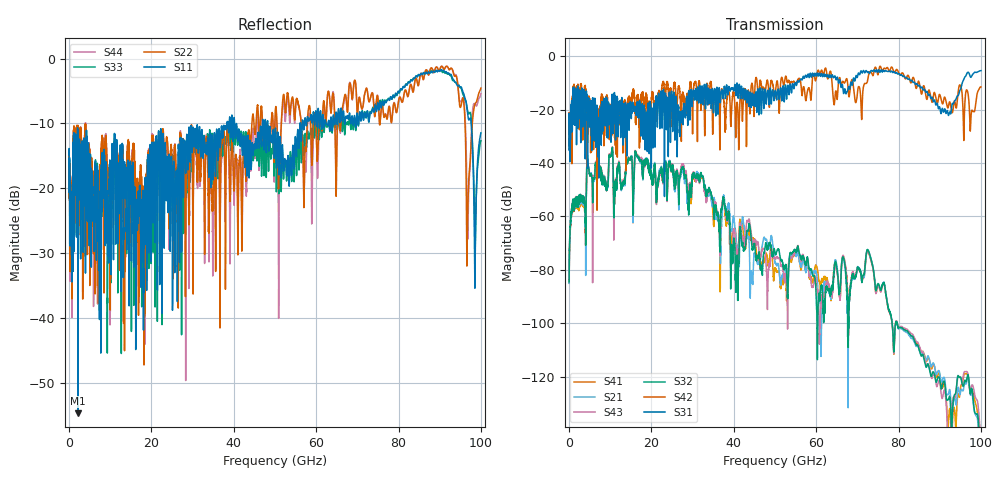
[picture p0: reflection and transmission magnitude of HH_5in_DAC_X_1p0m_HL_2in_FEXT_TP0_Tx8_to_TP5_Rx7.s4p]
# GHz S RI R 45
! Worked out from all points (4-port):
!   4000 points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, 25 MHz to 100 GHz, reference 45 ohm
!   strongest paths, dB at 25 MHz, 25.02 GHz, 50.02 GHz, 75.03 GHz, 100 GHz:
!     S31: -22.2, -15.3, -12.9, -5.7, -5.4
!     S42: -22.0, -22.6, -14.7, -7.0, -11.5
!     S32: -84.5, -41.9, -73.7, -85.2, -154.6
!     S43: -84.3, -41.7, -75.9, -85.9, -143.4
!     S21: -85.1, -42.2, -77.1, -85.1, -151.0
!     S41: -85.0, -42.2, -79.6, -85.8, -156.0
!   lowest |S11| = -54.7 dB at 2.2 GHz (marker M1), VSWR 1.00, Z = 44.9 - j0.0959 ohm
!   |S11| at or under -10 dB: start of sweep to 38.36 GHz; 40.2 GHz to 46.98 GHz (6.777 GHz wide, 15.5 % of centre); 48.27 GHz to 56.1 GHz (7.833 GHz wide, 15 % of centre)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
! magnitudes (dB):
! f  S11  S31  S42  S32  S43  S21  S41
! 25 MHz  -14.8  -22.2  -22.0  -84.5  -84.3  -85.1  -85.0
! 2.2 GHz  -54.7  -26.7  -23.1  -54.4  -54.5  -55.1  -56.0
! 16.45 GHz  -21.7  -18.6  -18.4  -37.1  -36.8  -37.2  -36.8
! 32.3 GHz  -11.1  -11.2  -13.3  -45.2  -45.4  -45.4  -45.8
! 40.77 GHz  -10.8  -10.2  -17.6  -76.4  -73.4  -72.4  -71.8
! 96.9 GHz  -9.0  -6.0  -14.2  -119.4  -119.3  -120.1  -120.1
! 100 GHz  -11.4  -5.4  -11.5  -154.6  -143.4  -151.0  -156.0
